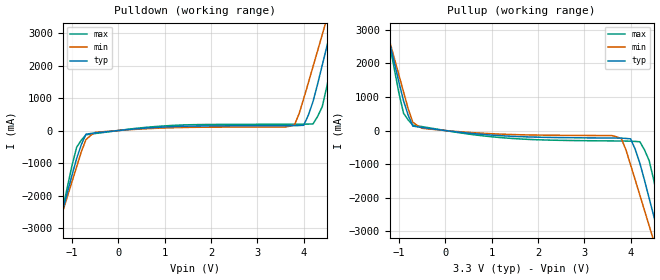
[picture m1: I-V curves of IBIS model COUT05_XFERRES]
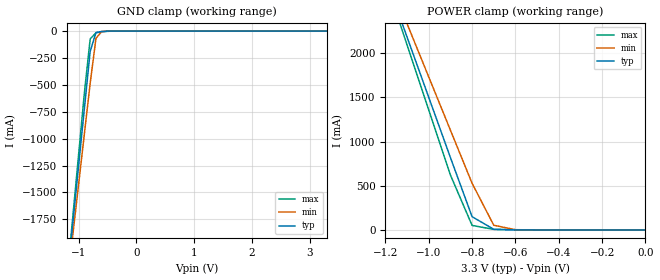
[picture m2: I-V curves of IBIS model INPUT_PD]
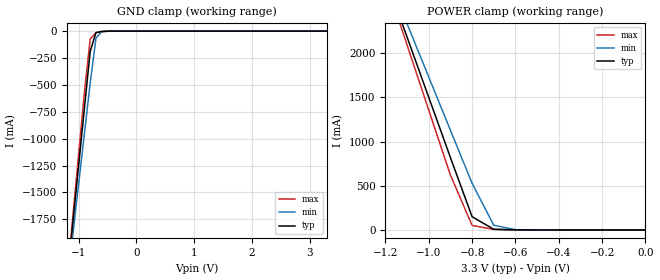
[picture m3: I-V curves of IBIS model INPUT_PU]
|   This file is an IBIS representation of the   |
|   Integrated Circuit Systems, Inc.   |
|   ICS87973I-147   |
[IBIS Ver]   3.2
[File name]   87973i-147_3v3.ibs
[File Rev]   0.0
[Date]   25 Aug 2005 | Last modified
|   09 Jan 2003 | Generated
[Source] Originated at Integrated Circuit Systems, Inc.
[Disclaimer]
(C) Copyright Integrated Circuit Systems, Inc. 1997
   All rights reserved
ICS hereby grants the user of this IBIS model a non-exclusive,
nontransferable license to use this IBIS model under the following terms.
Before using this IBIS model, the user should read this license.
If the user does not accept these terms,  the IBIS model should be
returned to ICS within 30 days.
   The user is granted this license only to use the IBIS model and
is not granted rights to sell, load, rent, lease or license the IBIS
model in whole or in part, or in modified form to anyone other than
user. User may modify the IBIS model to suit its specific
applications but rights to derivative works and such modifications
shall belong to ICS.
   This IBIS model is provided on an "AS IS" basis and ICS makes
absolutely no warranty with respect to the information contained
herein. ICS DISCLAIMS AND CUSTOMER WAIVES ALL WARRANTIES, EXPRESS
OR IMPLIED, INCLUDING WARRANTIES OF MERCHANTABILITY OR FITNESS FOR
A PARTICULAR PURPOSE. The entire risk as to quality and performance
is with the Customer. ACCORDINGLY, IN NO EVENT SHALL THE COMPANY BE
LIABLE FOR ANY DAMAGES, WHETHER IN CONTRACT OR TORT,INCLUDING ANY
LOST PROFITS OR OTHER INCIDENTAL, CONSEQUENTIAL, EXEMPLARY, OR
PUNITIVE DAMAGES ARISING OUT OF THE USE OR APPLICATION OF THE IBIS
model provided in this package. Further, ICS reserves the right to
make changes without notice to any product herein to improve
reliability, function, or design. ICS does not convey any license
under patent rights or any other intellectual property rights,
including those of third parties.
   ICS is not obligated to provide maintenance or support
for the licensed IBIS model.
[Copyright]   Copyright 2005 by Integrated Circuit Systems, Inc.
[Component]   ICS87973I-147
[Manufacturer] Integrated Circuit Systems, Inc.
[Package]
|LQFP 52 Pin
|   typ   min   max
R_pkg   52.85m   52.5m   53.2m
L_pkg   3.26nH   2.86nH   3.66nH
C_pkg   0.487pF   0.443pF   0.53pF
[Pin] signal_name   model_name
1   GNDI   GND
2   nMR/OE   INPUT_PU
|3 nc
|4 nc
5   FSEL_FB2   INPUT_PU
6   PLL_SEL   INPUT_PU
7   REF_SEL   INPUT_PU
8   CLK_SEL   INPUT_PU
9   CLK0   INPUT_PU
10   CLK1   INPUT_PU
11   CLK   INPUT_PD
|12   nCLK
13   VDDA   POWER
14   INV_CLK   INPUT_PU
15   GNDDO   GND
16   QC3   COUT05_XFERRES
17   VDDO   POWER
18   QC2   COUT05_XFERRES
19   FSEL_C1   INPUT_PU
20   FSEL_C0   INPUT_PU
21   QC1   COUT05_XFERRES
22   VDDO   POWER
23   QC0   COUT05_XFERRES
24   GNDO   GND
25   LOCK   COUT05_XFERRES
26   FSEL_FB1   INPUT_PU
27   FSEL_FB0   INPUT_PU
28   VDD   POWER
29   QFB   COUT05_XFERRES
30   GNDO   GND
31   EXT_FB   INPUT_PU
32   QB3   COUT05_XFERRES
33   VDDO   POWER
34   QB2   COUT05_XFERRES
35   GNDO   GND
36   QB1   COUT05_XFERRES
37   VDDO   POWER
38   QB0   COUT05_XFERRES
39   GNDO   GND
40   FSEB_B1   INPUT_PU
41   FSEL_B0   INPUT_PU
42   FSEL_A1   INPUT_PU
43   FSEL_A0   INPUT_PU
44   QA3   COUT05_XFERRES
45   VDDO   POWER
46   QA2   COUT05_XFERRES
47   GNDO   GND
48   QA1   COUT05_XFERRES
49   VDDO   POWER
50   QA0   COUT05_XFERRES
51   GNDO   GND
52   VCO_SEL   INPUT_PU
| Models and submodels in the file (3): COUT05_XFERRES (Output), INPUT_PD (Input), INPUT_PU (Input)
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|   ICS87973I-147 3.3V Clock Drive Model
| This model is suitable for all output pins on the
|  ICS87973I-147
[Model]   COUT05_XFERRES
Model_type   Output
Polarity   Non-Inverting
|   typ   min   max
C_comp   2pF   1.5pF   2.5pF
|   typ   min   max
[Voltage range]  3.3V   3.15V   3.45V
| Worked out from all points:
|   slope of the pulldown table from 0 to 0.495 V, typ, clamps not added: 7.71 ohm
|   slope of the pullup table from 0 to 0.495 V, typ, clamps not added: 6.44 ohm
[pulldown]
|Voltage   I (typ)   I (min)   I (max)
-3.3V     -13.74A    -12.12A    -16.25A
-1.4V     -3.526A    -3.407A    -3.72A
-1.3V     -2.987A    -2.948A    -3.058A
-900mV    -857.7mA   -1.112A    -513.9mA
-700mV    -114.2mA   -281.1mA   -130.4mA
3.8V      149.8mA    170.1mA    194.9mA
4V        161.9mA    982.2mA    196.3mA
4.2V      887.5mA    1.963A     202.2mA
4.4V      2.009A     2.952A     734.1mA
4.6V      3.173A     3.944A     2.074A
4.8V      4.339A     4.937A     3.509A
6.6V      15.05A     14.04A     16.69A
[pullup]
|Voltage   I (typ)   I (min)   I (max)
-3.3V     15.02A     13.23A     17.78A
-1.3V     3.212A     3.164A     3.296A
-900mV    885.7mA    1.151A     514.2mA
-700mV    133mA      248.7mA    161.5mA
3.6V      -223.7mA   -151.5mA   -310mA
3.8V      -226.2mA   -242.1mA   -312.1mA
4V        -247.6mA   -1.022A    -317.2mA
4.3V      -1.48A     -2.38A     -576.5mA
4.5V      -2.547A    -3.289A    -1.474A
4.6V      -3.081A    -3.743A    -2.13A
4.8V      -4.149A    -4.654A    -3.444A
6.6V      -13.78A    -12.87A    -15.26A
[Ramp]
|   typ   min   max
dV/dt_r   1.98/0.6n   1.98/0.80n   1.98/0.4n
dV/dt_f   1.98/0.6n   1.98/0.80n   1.98/0.4n
[Model]   INPUT_PD
Model_type   Input
Polarity   Non-Inverting
Vinl = 1.4V
Vinh = 1.85V
|   typ   min   max
C_comp   2pF   1.5pF   2.5pF
|   typ   min   max
[Voltage range]  3.3V   3.15V   3.45V
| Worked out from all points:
|   GND clamp passes 1 mA (typ) near -0.51 V on its own axis
|   POWER clamp passes 1 mA (typ) near -0.60 V on its own axis
[GND_clamp]
|Voltage I(typ)   I(min)   I(max)
-3.3V     -13.52A    -12.28A    -14.38A
-1.2V     -2.314A    -2.362A    -2.296A
-1.1V     -1.782A    -1.891A    -1.721A
-1V       -1.25A     -1.422A    -1.146A
-900mV    -718.5mA   -952.6mA   -572.1mA
-800mV    -188.2mA   -484.5mA   -72.95mA
-700mV    -13.66mA   -66.68mA   -15.82mA
-600mV    -3.044mA   -4.415mA   -6.968mA
-500mV    -658.9uA   -400.5uA   -2.169mA
3.3V      64.58uA    64.62uA    64.6uA
[POWER_clamp]
|Voltage   I(typ)   I(min)   I(max)
-3.3V     17.27A     15.67A     18.38A
-1.2V     2.866A     2.938A     2.832A
-1.1V     2.183A     2.334A     2.094A
-1V       1.501A     1.732A     1.358A
-900mV    819.8mA    1.13A      621.9mA
-800mV    150.3mA    528.4mA    51.58mA
-700mV    7.809mA    53.45mA    6.607mA
-600mV    968.4uA    3.161mA    1.955mA
0V        64.58uA    61.35uA    67.83uA
[Model]   INPUT_PU
Model_type   Input
Polarity   Non-Inverting
Vinl = 1.4V
Vinh = 1.85V
|   typ   min   max
C_comp   2pF   1.5pF   2.5pF
|   typ   min   max
[Voltage range]  3.3V   3.15V   3.45V
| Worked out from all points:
|   GND clamp passes 1 mA (typ) near -0.51 V on its own axis
|   POWER clamp passes 1 mA (typ) near -0.60 V on its own axis
[GND_clamp]
|Voltage   I(typ)   I(min)   I(max)
-3.3V     -13.52A    -12.28A    -14.38A
-1.2V     -2.314A    -2.362A    -2.296A
-1.1V     -1.782A    -1.891A    -1.721A
-1V       -1.25A     -1.422A    -1.146A
-900mV    -718.6mA   -952.7mA   -572.2mA
-800mV    -188.2mA   -484.6mA   -73.02mA
-700mV    -13.72mA   -66.74mA   -15.89mA
-600mV    -3.109mA   -4.477mA   -7.036mA
-500mV    -723.5uA   -462.1uA   -2.236mA
3.3V      3.748nA    2.972uA    -2.918uA
[POWER_clamp]
|Voltage   I(typ)   I(min)   I(max)
-3.3V     17.27A     15.67A     18.38A
-1.2V     2.866A     2.938A     2.832A
-1.1V     2.183A     2.334A     2.094A
-1V       1.501A     1.732A     1.358A
-900mV    819.7mA    1.129A     621.8mA
-800mV    150.2mA    528.4mA    51.51mA
-700mV    7.744mA    53.39mA    6.54mA
-600mV    903.9uA    3.099mA    1.887mA
0V        3.748nA    2.31nA     19.96nA
